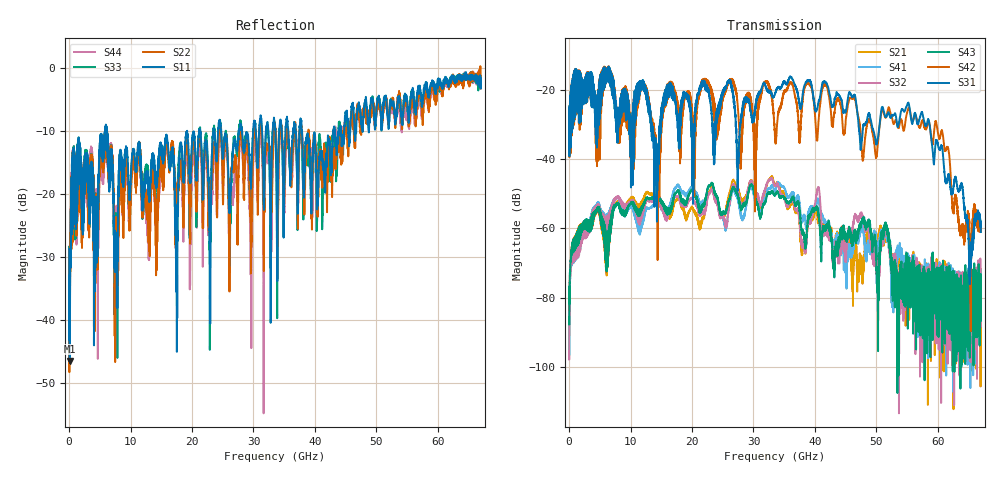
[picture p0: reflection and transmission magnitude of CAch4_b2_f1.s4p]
!Agilent Technologies,N5247A,US51170199,A.09.90.13
!Agilent N5247A: A.09.90.13
!Date: Thursday, October 18, 2018 11:54:46
!Correction: S11(Full 4 Port(1,2,3,4))
!S12(Full 4 Port(1,2,3,4))
!S13(Full 4 Port(1,2,3,4))
!S14(Full 4 Port(1,2,3,4))
!S21(Full 4 Port(1,2,3,4))
!S22(Full 4 Port(1,2,3,4))
!S23(Full 4 Port(1,2,3,4))
!S24(Full 4 Port(1,2,3,4))
!S31(Full 4 Port(1,2,3,4))
!S32(Full 4 Port(1,2,3,4))
!S33(Full 4 Port(1,2,3,4))
!S34(Full 4 Port(1,2,3,4))
!S41(Full 4 Port(1,2,3,4))
!S42(Full 4 Port(1,2,3,4))
!S43(Full 4 Port(1,2,3,4))
!S44(Full 4 Port(1,2,3,4))
!S4P File: Measurements: <S11,S12,S13,S14>,
!<S21,S22,S23,S24>,
!<S31,S32,S33,S34>,
!<S41,S42,S43,S44>:
# Hz S  dB  R 50
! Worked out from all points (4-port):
!   6701 points, 10 MHz to 67 GHz, reference 50 ohm
!   strongest paths, dB at 10 MHz, 16.76 GHz, 33.51 GHz, 50.25 GHz, 67 GHz:
!     S31: -30.6, -22.5, -21.2, -33.9, -61.1
!     S42: -30.7, -20.2, -33.3, -35.2, -59.5
!     S43: -85.5, -52.8, -50.5, -76.6, -78.8
!     S32: -95.4, -52.9, -47.8, -75.1, -88.4
!     S41: -83.7, -50.7, -49.1, -66.3, -76.7
!     S21: -86.7, -54.8, -47.5, -65.1, -80.0
!   lowest |S11| = -46.5 dB at 99.99 MHz (marker M1), VSWR 1.01, Z = 49.6 - j0.216 ohm
!   |S11| at or under -10 dB: start of sweep to 5.851 GHz; 6.182 GHz to 21.18 GHz (15 GHz wide, 110 % of centre); 37.9 GHz to 43 GHz (5.101 GHz wide, 12.6 % of centre)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
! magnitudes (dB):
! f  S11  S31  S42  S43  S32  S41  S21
! 10 MHz  -28.8  -30.6  -30.7  -85.5  -95.4  -83.7  -86.7
! 99.99 MHz  -46.5  -26.8  -27.0  -76.5  -79.4  -79.3  -76.9
! 4.579 GHz  -21.6  -23.5  -23.9  -54.2  -53.2  -52.7  -54.5
! 14.43 GHz  -16.1  -41.7  -40.9  -51.0  -51.7  -52.6  -50.6
! 32.81 GHz  -38.3  -20.5  -20.5  -49.8  -45.6  -48.3  -45.3
! 55.12 GHz  -6.7  -23.9  -25.9  -70.5  -72.7  -68.9  -70.7
! 67 GHz  -3.3  -61.1  -59.5  -78.8  -88.4  -76.7  -80.0
